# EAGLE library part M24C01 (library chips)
1K I2C™ Serial EEPROM
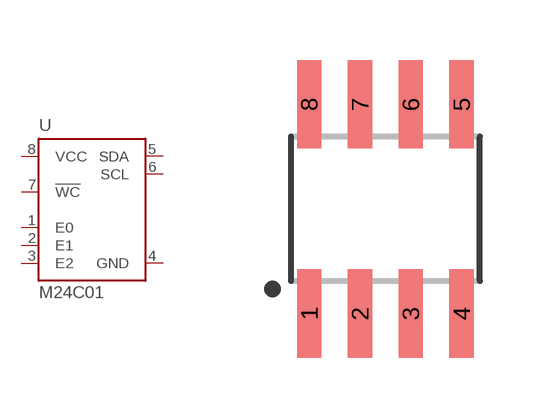
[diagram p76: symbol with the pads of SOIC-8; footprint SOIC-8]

Designator prefix U

## M24C01WMN (DIGIKEY: 497-8631-1-ND)  [SOIC-8]
1  E0
2  E1
3  E2
4  GND
5  SDA
6  SCL
7  !WC
8  VCC

## Footprint SOIC-8 (pad centres in mm)
smd 0.61 x 2.21: 1 -1.905,-2.616; 2 -0.635,-2.616; 3 0.635,-2.616; 4 1.905,-2.616; 5 1.905,2.616; 6 0.635,2.616; 7 -0.635,2.616; 8 -1.905,2.616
